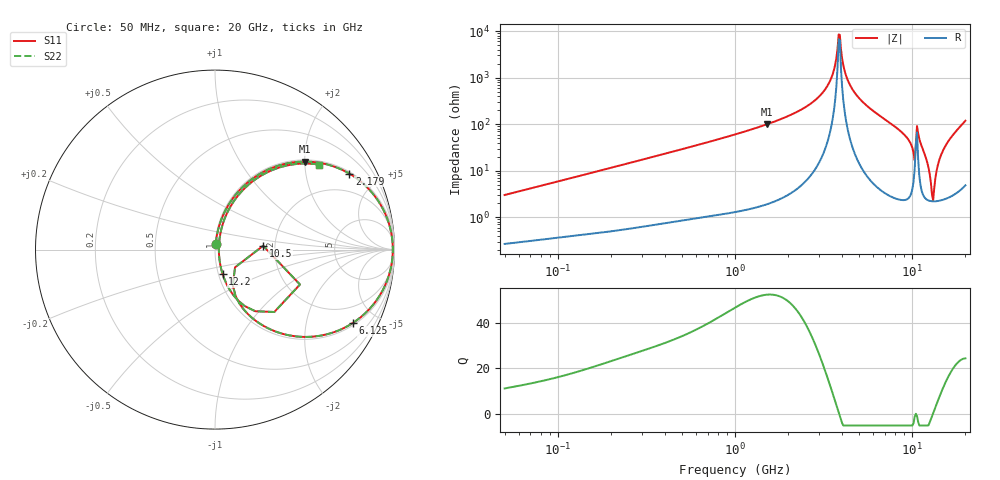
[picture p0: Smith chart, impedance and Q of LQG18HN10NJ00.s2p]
!Murata Part Number: LQG18HN10NJ00
!These Parameters are Measured in Series Mode Connection
!  o--[Z]--o
!Port1  Port2
!  o-------o
!Freq. Start=50[MHz] Stop=20[GHz], 401[Steps]
# Hz S RI R 50
!Freq.(Hz) S11(Real) S11(Imag) S21(Real) S21(Imag) S12(Real) S12(Imag) S22(Real) S22(Imag)
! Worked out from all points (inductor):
!   401 points, 50 MHz to 20 GHz, reference 50 ohm
!   read as one part in series: L = 9.46 nH near 51.52 MHz
!   highest Q = 52.3 at 1.521 GHz (marker M1), where L = 10.5 nH
!   self-resonance near 3.85 GHz
!   S11 on the Smith chart (normalised r, x): 50 MHz: 1.01, +0.06; 2.179 GHz: 1.08, +3.49; 6.125 GHz: 1.10, -3.69; 10.5 GHz: 1.73, +0.08; 12.2 GHz: 1.05, -0.29; 20 GHz: 1.10, +2.37
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5e7  0.00356 0.0298  0.9964 -0.0298  0.9964 -0.0298  0.00356 0.0298
1.364002e8  0.0104 0.0784  0.9896 -0.0784  0.9896 -0.0784  0.0104 0.0784
3.721004e8  0.0502 0.2024  0.9498 -0.2024  0.9498 -0.2024  0.0502 0.2024
1e9  0.2701 0.4334  0.7299 -0.4334  0.7299 -0.4334  0.2701 0.4334
1.521052e9  0.5 0.4905  0.5 -0.4905  0.5 -0.4905  0.5 0.4905
2.179053e9  0.7486 0.4232  0.2514 -0.4232  0.2514 -0.4232  0.7486 0.4232
2.728004e9  0.8879 0.3009  0.1121 -0.3009  0.1121 -0.3009  0.8879 0.3009
3.415248e9  0.976 0.1202  0.024 -0.1202  0.024 -0.1202  0.976 0.1202
3.792786e9  0.9903 0.0216  0.0097 -0.0216  0.0097 -0.0216  0.9903 0.0216
3.908127e9  0.9907 -0.00752  0.00933 0.00752  0.00933 0.00752  0.9907 -0.00752
4.149438e9  0.9861 -0.0665  0.0139 0.0665  0.0139 0.0665  0.9861 -0.0665
4.472136e9  0.9698 -0.1405  0.0302 0.1405  0.0302 0.1405  0.9698 -0.1405
6.125241e9  0.7667 -0.4096  0.2333 0.4096  0.2333 0.4096  0.7667 -0.4096
7.442007e9  0.5398 -0.4853  0.4602 0.4853  0.4602 0.4853  0.5398 -0.4853
9.178299e9  0.2463 -0.4102  0.7537 0.4102  0.7537 0.4102  0.2463 -0.4102
1.004137e10  0.1149 -0.2594  0.8851 0.2594  0.8851 0.2594  0.1149 -0.2594
1.050288e10  0.2684 0.0212  0.7316 -0.0212  0.7316 -0.0212  0.2684 0.0212
1.098561e10  0.2241 -0.3433  0.7759 0.3433  0.7759 0.3433  0.2241 -0.3433
1.220001e10  0.0422 -0.1357  0.9578 0.1357  0.9578 0.1357  0.0422 -0.1357
1.314879e10  0.0216 0.0072  0.9784 -0.0072  0.9784 -0.0072  0.0216 0.0072
1.504638e10  0.0935 0.2522  0.9065 -0.2522  0.9065 -0.2522  0.0935 0.2522
2e10  0.5809 0.4734  0.4191 -0.4734  0.4191 -0.4734  0.5809 0.4734
